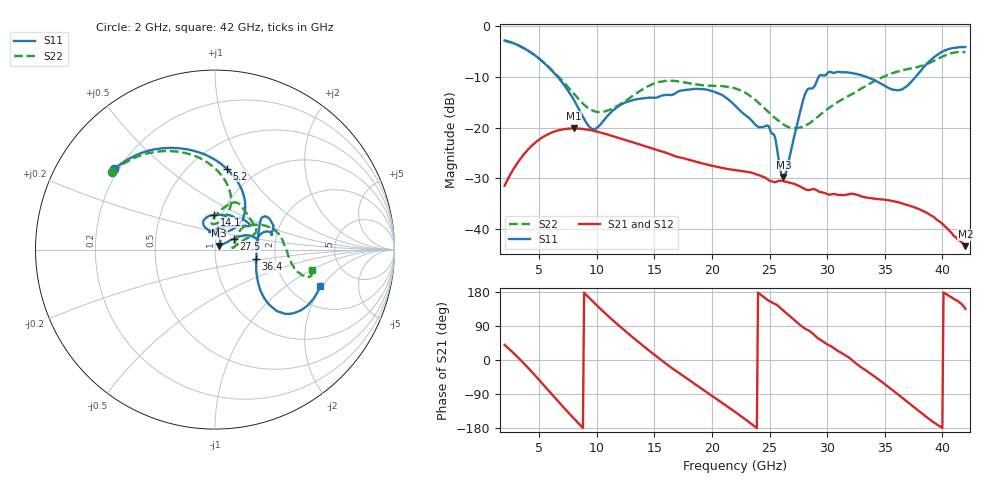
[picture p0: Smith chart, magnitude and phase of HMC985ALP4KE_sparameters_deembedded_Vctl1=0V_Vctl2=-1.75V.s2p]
!s2p File: Measurements: S11, S21, S12, S22
# GHz S dB R 50.0
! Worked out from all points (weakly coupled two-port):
!   401 points, 2 GHz to 42 GHz, reference 50 ohm
!   highest |S21| = -20.19 dB at 8 GHz (marker M1); lowest = -43.4 dB at 42 GHz (marker M2)
!   lowest |S11| = -29.7 dB at 26.2 GHz (marker M3), VSWR 1.07, Z = 52.4 + j2.34 ohm
!   |S11| at or under -10 dB: 6.587 GHz to 29.27 GHz (22.68 GHz wide, 127 % of centre); 33.36 GHz to 37.69 GHz (4.334 GHz wide, 12.2 % of centre)
!   |S22| runs from -20.2 to -2.9 dB; largest |S21 - S12| = 0.0002
!   S11 on the Smith chart (normalised r, x): 2 GHz: 0.18, +0.34; 5.2 GHz: 0.74, +0.84; 14.1 GHz: 0.92, +0.37; 27.5 GHz: 1.22, +0.15; 36.4 GHz: 1.58, -0.18; 42 GHz: 2.90, -1.91
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2  -2.86 141.4  -31.48 39.7  -31.48 39.7  -2.88 142.8
3.6  -4.28 112.0  -25.50 -6.7  -25.50 -6.7  -4.33 115.4
5.2  -6.83 81.8  -22.06 -59.6  -22.07 -59.6  -6.81 90.5
8  -14.51 46.6  -20.19 -154.0  -20.19 -154.0  -13.34 70.6
8.7  -17.47 52.1  -20.27 -176.2  -20.27 -176.3  -15.09 75.2
9.8  -20.32 87.3  -20.69 150.2  -20.69 150.2  -16.82 88.5
12  -15.64 113.5  -22.12 88.7  -22.12 88.7  -15.47 94.3
14.1  -14.22 91.1  -23.60 35.5  -23.60 35.5  -12.31 77.3
15.4  -13.94 73.1  -24.55 4.6  -24.55 4.6  -11.05 69.1
19.4  -12.52 34.3  -27.20 -81.9  -27.20 -81.9  -11.73 38.9
22  -15.66 52.3  -28.39 -136.8  -28.39 -136.8  -12.29 22.2
25  -20.12 98.3  -30.48 155.2  -30.49 155.2  -17.18 15.0
26.2  -29.75 43.4  -30.57 130.1  -30.57 130.1  -19.39 7.6
27.5  -18.36 30.0  -31.45 96.1  -31.46 96.1  -20.07 6.9
28.1  -13.33 20.9  -32.16 82.3  -32.18 82.4  -19.63 11.9
28.7  -12.29 13.0  -32.16 71.1  -32.17 71.1  -18.77 18.4
31  -9.07 23.3  -33.27 22.9  -33.30 22.8  -14.87 38.0
33.3  -9.95 34.3  -33.74 -26.3  -33.76 -26.3  -11.91 32.6
35.4  -12.27 12.2  -34.35 -73.1  -34.37 -73.0  -9.55 21.3
36.4  -12.58 -13.0  -34.89 -96.9  -34.87 -97.0  -8.78 14.5
39.5  -5.81 -43.3  -38.12 -169.4  -38.06 -169.6  -6.57 -14.1
42  -4.14 -19.0  -43.36 135.0  -43.32 134.9  -5.14 -11.8
